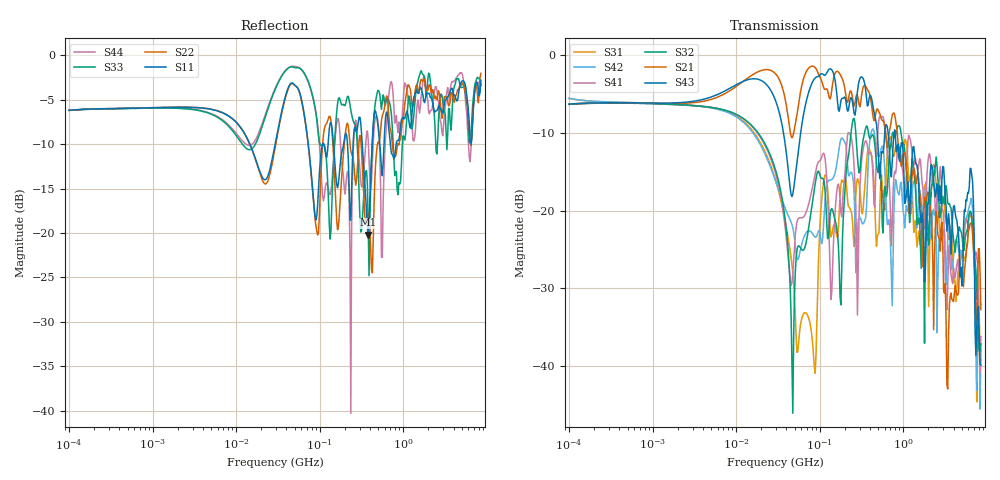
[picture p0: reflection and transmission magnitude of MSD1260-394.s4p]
# MHz S MA R 50
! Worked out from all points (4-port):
!   498 points, 100 kHz to 8.5 GHz, reference 50 ohm
!   strongest paths, dB at 100 kHz, 1.698 MHz, 29.49 MHz, 500.7 MHz, 8.5 GHz:
!     S43: -6.4, -6.2, -5.9, -12.0, -39.8
!     S21: -6.4, -6.3, -2.4, -7.2, -32.7
!     S32: -6.4, -6.4, -14.8, -15.1, -37.1
!     S41: -6.4, -6.4, -15.2, -9.3, -36.2
!     S42: -5.6, -6.4, -16.2, -12.9, -37.7
!     S31: -5.6, -6.4, -16.0, -23.0, -39.3
!   lowest |S11| = -20.2 dB at 380.6 MHz (marker M1), VSWR 1.22, Z = 58.9 - j5.94 ohm
!   |S11| at or under -10 dB: 323.1 MHz to 424.4 MHz (101.3 MHz wide, 27.1 % of centre); 523.4 MHz to 588.4 MHz (65.01 MHz wide, 11.7 % of centre); 701.2 MHz to 822.8 MHz (121.7 MHz wide, 16 % of centre)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
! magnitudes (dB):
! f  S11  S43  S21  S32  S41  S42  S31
! 100 kHz  -6.2  -6.4  -6.4  -6.4  -6.4  -5.6  -5.6
! 15.92 MHz  -10.9  -3.1  -2.5  -9.3  -9.4  -10.1  -9.9
! 47.64 MHz  -3.1  -17.9  -10.5  -46.0  -28.0  -22.2  -28.0
! 380.6 MHz  -20.2  -6.4  -4.7  -9.8  -12.5  -13.9  -12.1
! 3.409 GHz  -4.7  -21.5  -42.9  -19.0  -29.7  -23.3  -23.1
! 6.462 GHz  -10.0  -14.6  -21.6  -20.2  -20.8  -18.4  -20.4
! 8.5 GHz  -2.8  -39.8  -32.7  -37.1  -36.2  -37.7  -39.3
